(* Logix 5000 AddOnInstructionDefinition export Banner_EZAK2_Param_v4; software revision 33.00; part 3 of 3 *)
(* tags used below, declared in another part *)
   EZAK2 : Banner_EZAK2_v4;
   Port_Data : Banner_IOL_Port_v4;
   Port : DINT;
   Local_Control : DINT;
   Command_Being_Processed : BOOL;
   Update_Archive : BOOL;
   Index_Write_Inprocess : INT;
   Inprocess_Index : DINT;
(* Banner_EZAK2_Param_v4, continued *)

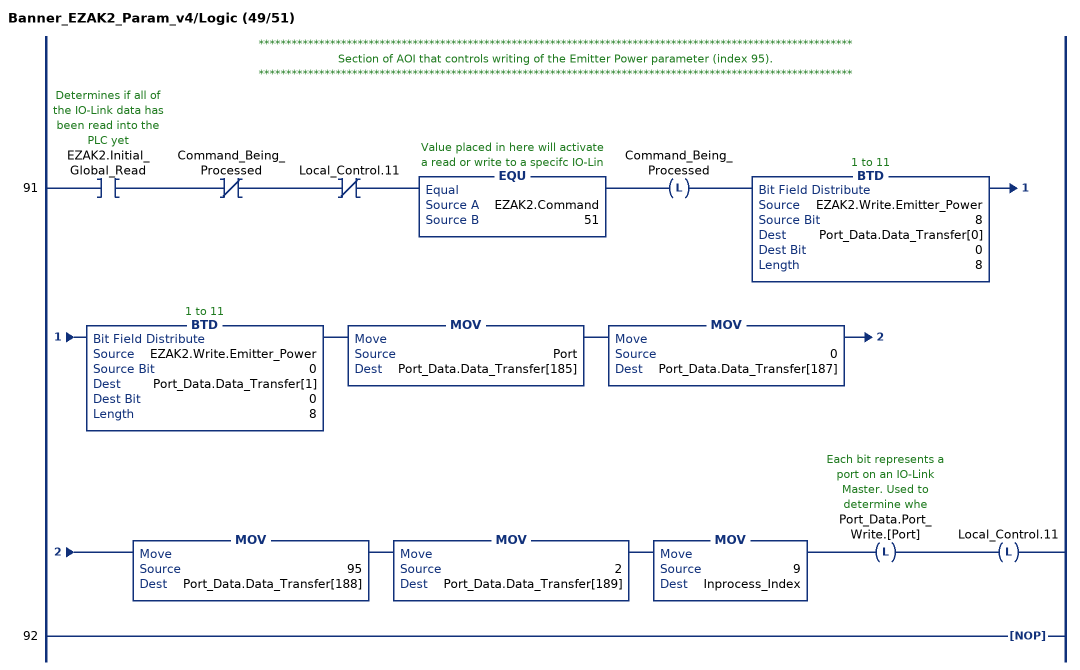
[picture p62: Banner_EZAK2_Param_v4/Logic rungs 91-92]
   // ************************************************************************************************************
   // Section of AOI that controls writing of the Emitter Power parameter (index 95).
   // ************************************************************************************************************
   91: XIC(EZAK2.Initial_Global_Read)XIO(Command_Being_Processed)XIO(Local_Control.11)EQU(EZAK2.Command,51)OTL(Command_Being_Processed)BTD(EZAK2.Write.Emitter_Power,8,Port_Data.Data_Transfer[0],0,8)BTD(EZAK2.Write.Emitter_Power,0,Port_Data.Data_Transfer[1],0,8)MOV(Port,Port_Data.Data_Transfer[185])MOV(0,Port_Data.Data_Transfer[187])MOV(95,Port_Data.Data_Transfer[188])MOV(2,Port_Data.Data_Transfer[189])MOV(9,Inprocess_Index)OTL(Port_Data.Port_Write.[Port])OTL(Local_Control.11);
   92: NOP();
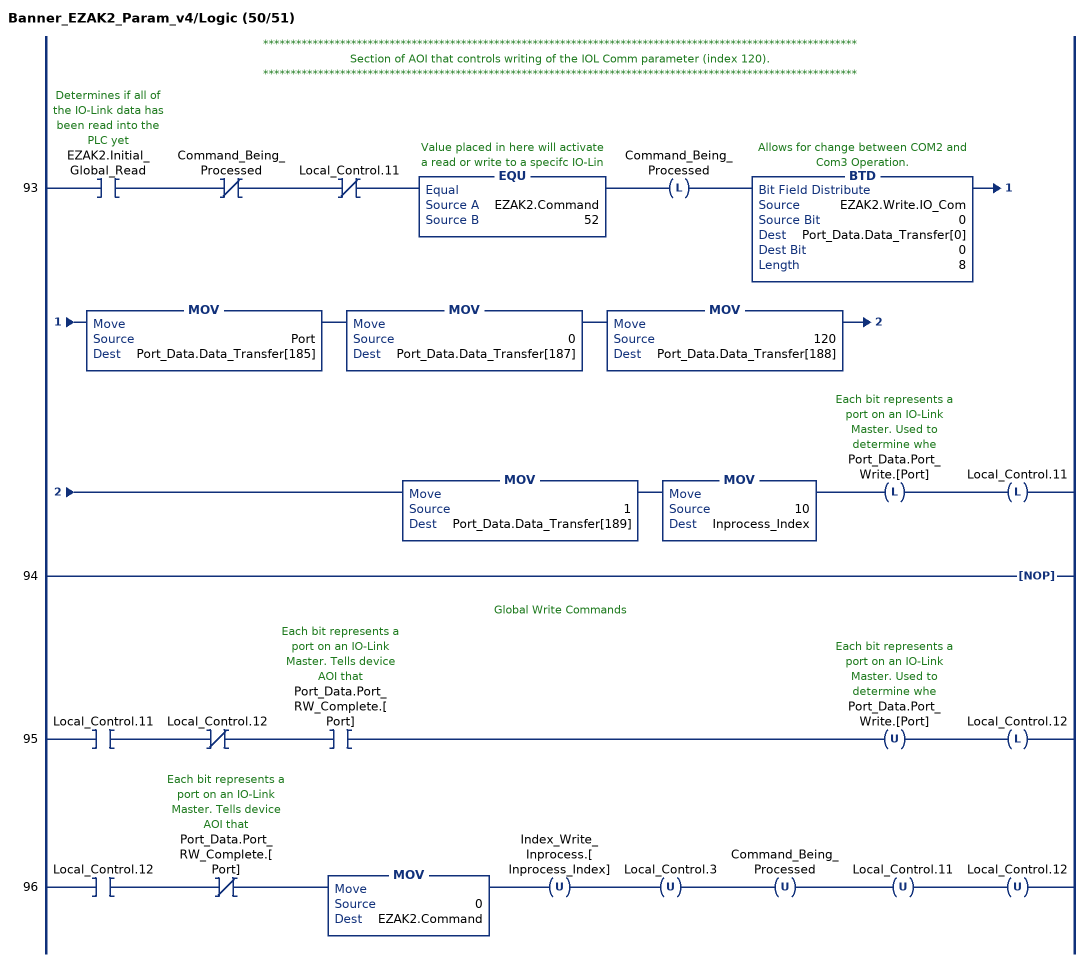
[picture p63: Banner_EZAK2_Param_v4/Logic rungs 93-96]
   // ************************************************************************************************************
   // Section of AOI that controls writing of the IOL Comm parameter (index 120).
   // ************************************************************************************************************
   93: XIC(EZAK2.Initial_Global_Read)XIO(Command_Being_Processed)XIO(Local_Control.11)EQU(EZAK2.Command,52)OTL(Command_Being_Processed)BTD(EZAK2.Write.IO_Com,0,Port_Data.Data_Transfer[0],0,8)MOV(Port,Port_Data.Data_Transfer[185])MOV(0,Port_Data.Data_Transfer[187])MOV(120,Port_Data.Data_Transfer[188])MOV(1,Port_Data.Data_Transfer[189])MOV(10,Inprocess_Index)OTL(Port_Data.Port_Write.[Port])OTL(Local_Control.11);
   94: NOP();
   // Global Write Commands
   95: XIC(Local_Control.11)XIO(Local_Control.12)XIC(Port_Data.Port_RW_Complete.[Port])OTU(Port_Data.Port_Write.[Port])OTL(Local_Control.12);
   96: XIC(Local_Control.12)XIO(Port_Data.Port_RW_Complete.[Port])MOV(0,EZAK2.Command)OTU(Index_Write_Inprocess.[Inprocess_Index])OTU(Local_Control.3)OTU(Command_Being_Processed)OTU(Local_Control.11)OTU(Local_Control.12);
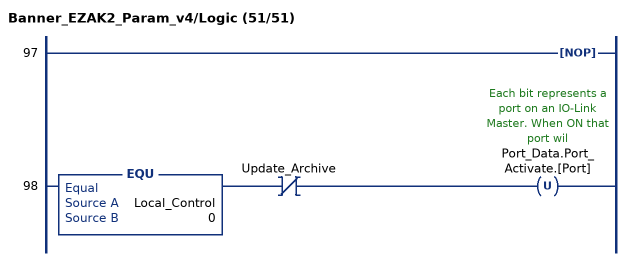
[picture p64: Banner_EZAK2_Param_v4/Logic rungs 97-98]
   97: NOP();
   98: EQU(Local_Control,0)XIO(Update_Archive)OTU(Port_Data.Port_Activate.[Port]);
END_ROUTINE
END_ADD_ON_INSTRUCTION
